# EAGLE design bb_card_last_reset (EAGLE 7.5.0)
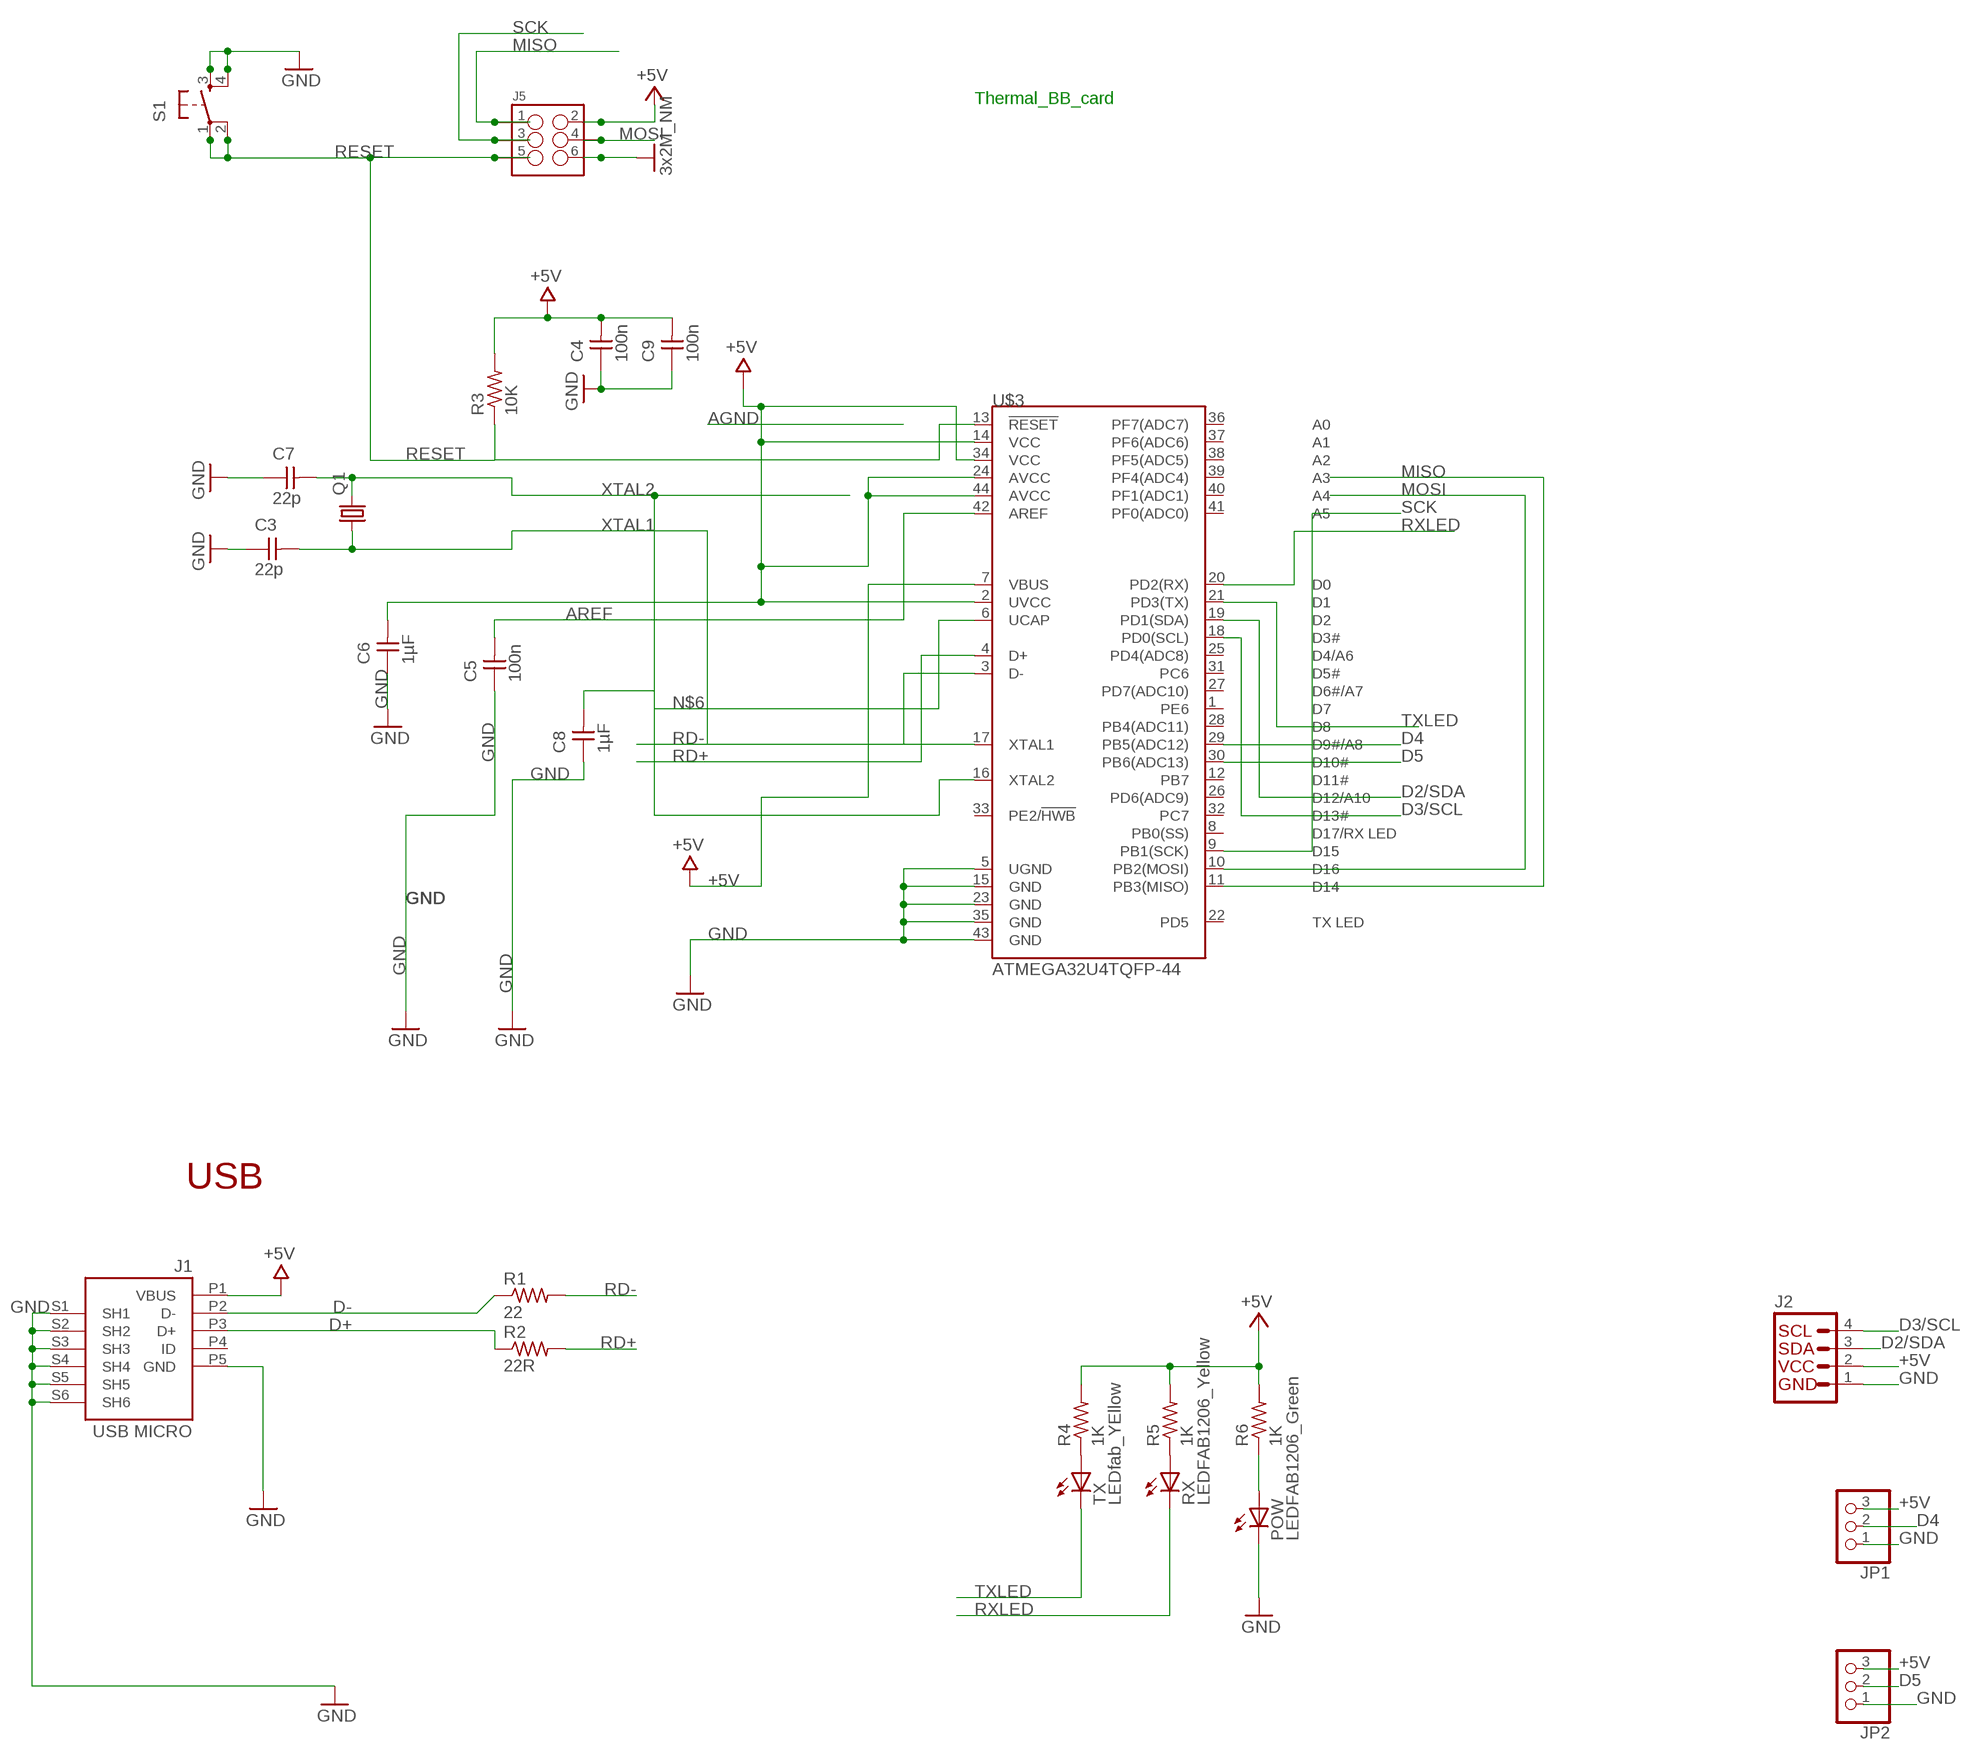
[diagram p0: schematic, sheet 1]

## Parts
C3  22p  CAP-UNPOLARIZEDFAB  [C1206FAB]
C4  100n  CAP-UNPOLARIZEDFAB  [C1206FAB]
C5  100n  CAP-UNPOLARIZEDFAB  [C1206FAB]
C6  1µF  CAP-UNPOLARIZEDFAB  [C1206FAB]
C7  22p  CAP-UNPOLARIZEDFAB  [C1206FAB]
C8  1µF  CAP-UNPOLARIZEDFAB  [C1206FAB]
C9  100n  CAP-UNPOLARIZEDFAB  [C1206FAB]
J1  USB MICRO  MYCON2_USB-MINI-B  [CON2_USB_MICRO_B_AT]
J2  I2C_STANDARD  [1X04]
J5  M03X2  [2X3_SMD]
JP1  PINHD-1X3  [1X03]
JP2  PINHD-1X3  [1X03]
POW  LEDFAB1206_Green  LEDFAB1206  [LED1206FAB]
Q1  CRYSTALHC49UP  [HC49UP]
R1  22  RES-US1206FAB  [R1206FAB]
R2  22R  RES-US1206FAB  [R1206FAB]
R3  10K  RES-US1206FAB  [R1206FAB]
R4  1K  RES-US1206FAB  [R1206FAB]
R5  1K  RES-US1206FAB  [R1206FAB]
R6  1K  RES-US1206FAB  [R1206FAB]
RX  LEDFAB1206_Yellow  LEDFAB1206  [LED1206FAB]
S1  6MM_SWITCH6MM_SWITCH  [6MM_SWITCH]
TX  LEDfab_YEllow  LEDFAB1206  [LED1206FAB]
U$3  ATMEGA32U4TQFP-44  [TQFP44]

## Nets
+5V [usbvcc]: C4.2 C6.2 C9.2 J1.P1(VBUS) J2.2 J5.2 JP1.3 JP2.3 R3.2 R4.2 R5.2 R6.2 U$3.2(UVCC) U$3.7(VBUS) U$3.14(VCC) U$3.24(AVCC) U$3.34(VCC) U$3.44(AVCC)
AREF [aref]: C5.2 U$3.42(AREF)
D2/SDA: J2.3 U$3.19(PD1(SDA))
D3/SCL: J2.4 U$3.18(PD0(SCL))
D4: JP1.2 U$3.29(PB5(ADC12))
D5: JP2.2 U$3.30(PB6(ADC13))
D+: J1.P3(D+) R2.1
D-: J1.P2(D-) R1.1
GND [gnd]: C3.1 C4.1 C5.1 C6.1 C7.1 C8.1 C9.1 J1.P5(GND) J1.S1(SH1) J1.S2(SH2) J1.S3(SH3) J1.S4(SH4) J1.S5(SH5) J1.S6(SH6) J2.1 J5.6 JP1.1 JP2.1 POW.2(C) S1.3(S) S1.4(S1) U$3.5(UGND) U$3.15(GND) U$3.23(GND) U$3.35(GND) U$3.43(GND) ; supply symbol labelled 3x2M_NM
MISO: J5.1 U$3.11(PB3(MISO))
MOSI: J5.4 U$3.10(PB2(MOSI))
N$1: R4.1 TX.1(A)
N$2: R5.1 RX.1(A)
N$3: POW.1(A) R6.1
N$6: C8.2 U$3.6(UCAP)
RD+: R2.2 U$3.4(D+)
RD-: R1.2 U$3.3(D-)
RESET: J5.5 R3.1 S1.1(P) S1.2(P1) U$3.13(!RESET)
RXLED: RX.2(C) U$3.20(PD2(RX))
SCK: J5.3 U$3.9(PB1(SCK))
TXLED: TX.2(C) U$3.21(PD3(TX))
XTAL1: C3.2 Q1.1 U$3.17(XTAL1)
XTAL2: C7.2 Q1.2 U$3.16(XTAL2)
Unconnected: J1.P4(ID) U$3.1(PE6) U$3.8(PB0(SS)) U$3.12(PB7) U$3.22(PD5) U$3.25(PD4(ADC8)) U$3.26(PD6(ADC9)) U$3.27(PD7(ADC10)) U$3.28(PB4(ADC11)) U$3.31(PC6) U$3.32(PC7) U$3.33(PE2/!HWB) U$3.36(PF7(ADC7)) U$3.37(PF6(ADC6)) U$3.38(PF5(ADC5)) U$3.39(PF4(ADC4)) U$3.40(PF1(ADC1)) U$3.41(PF0(ADC0))

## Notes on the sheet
- Thermal_BB_card
- USB

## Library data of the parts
C3-C9 = fab (1):CAP-UNPOLARIZED
J1 = SmartPrj:MYCON2_USB-MINI-B
J2 = SparkFun-Connectors:I2C_STANDARD: SparkFun has standardized on a pinout for all I2C based sensor breakouts. This pinout allows I2C boards to be plugged directly into the headers on Arduino Uno compatible boards, and to be daisy chained easily.
J5 = SparkFun-Connectors:M03X2: 2x3 .1" header. Shrouded, with keying- CONN-10681 SMT- CONN-11415 Pogo pins- HW-11044; PROD_ID: CONN-11290
JP1 JP2 = pinhead:PINHD-1X3: PIN HEADER
POW RX TX = fab (1):LED: LED
Q1 = crystal:CRYSTAL: CRYSTAL; OC_FARNELL: unknown; OC_NEWARK: unknown
R1-R6 = fab (1):RES-US: Resistor (US Symbol)
S1 = fab (1):6MM_SWITCH: OMRON SWITCH
U$3 = SparkFun-DigitalIC:ATMEGA32U4: Atmel 44-pin 8-bit Microcontroller with 32KBytes of ISP Flash and USB Controller

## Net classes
0 default: width 0.254 mm, drill 0.61 mm, clearance 0.254 mm
1 power: width 0.254 mm, drill 0.61 mm, clearance 0.254 mm
2 gnd: width 0.254 mm, drill 0.61 mm, clearance 0.254 mm
3 usbvcc: width 0.254 mm, drill 0.61 mm, clearance 0.254 mm
4 aref: width 0.254 mm, drill 0.61 mm, clearance 0.254 mm

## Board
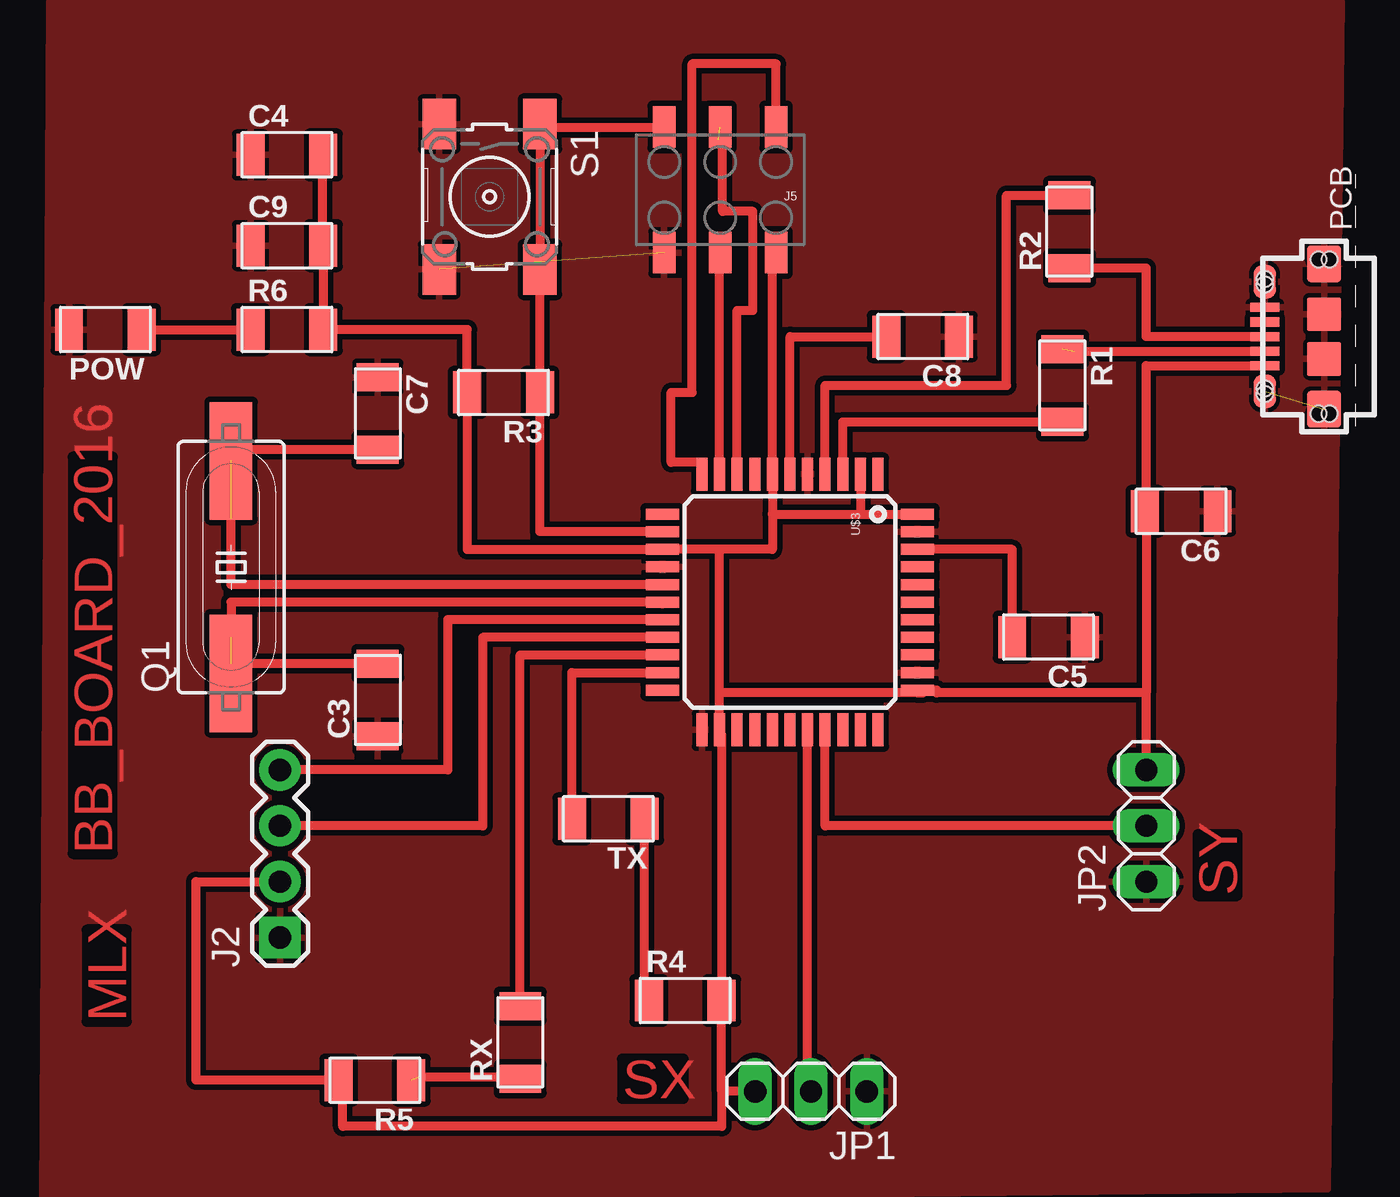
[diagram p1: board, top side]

No outline drawn. Coordinates in mm, seen from the top.
Copper layers (1*16): Top 0.018mm / dielectric 1.55mm / Bottom 0.018mm
Design rules "eC_2Layer_PClass6_BaseCopperO18_eCDefault *": minimum track width 0.15mm, minimum drill 0.35mm, track to track 0.01mm, track to pad 0.01mm, pad to pad 0.01mm, via to via 0.15mm, smd to smd 0mil, copper to edge 0.25mm, drill to drill 0.35mm, minimum pad ring 0.175mm, minimum via ring 0.125mm, stop-mask expansion 0mil, vias tented up to drill 0.45mm, thermal gap 0.2mm

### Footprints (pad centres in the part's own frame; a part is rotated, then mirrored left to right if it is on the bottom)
C1206FAB = smd 1.27 x 1.905: 1 -1.651,0; 2 1.651,0
CON2_USB_MICRO_B_AT = smd 0.406 x 1.346: P1 -1.321,2.692; P2 -0.66,2.692; P3 0,2.692; P4 0.66,2.692; P5 1.321,2.692 | smd 1.651 x 1.549: S1 -3.302,0; S2 3.302,0 | smd 1.524 x 1.016: S3 -2.489,2.692; S4 2.489,2.692 | smd 1.524 x 1.524: S5 -1.016,0; S6 1.016,0 | hole 0.7: -3.505,0.254; -3.505,-0.254; 3.505,0.254; 3.505,-0.254; -2.616,2.692; -2.362,2.692; 2.362,2.692; 2.616,2.692
1X04 = drill 1.016 pad 1.88 square: 1 0,0 | drill 1.016 pad 1.88: 2 2.54,0; 3 5.08,0; 4 7.62,0
2X3_SMD = smd 1.02 x 1.9: 1 -2.54,-2.85; 2 -2.54,2.85; 3 0,-2.85; 4 0,2.85; 5 2.54,-2.85; 6 2.54,2.85
1X03 = drill 1.016 long: 1 -2.54,0; 2 0,0; 3 2.54,0
LED1206FAB = smd 1.27 x 1.905: 1 -1.651,0; 2 1.651,0
HC49UP = smd 5.334 x 1.93: 1 -4.826,0; 2 4.826,0
R1206FAB = smd 1.27 x 1.905: 1 -1.651,0; 2 1.651,0
6MM_SWITCH = smd 2.286 x 1.524: 1 -3.302,2.286; 2 3.302,2.286; 3 -3.302,-2.286; 4 3.302,-2.286
TQFP44 = smd 1.5 x 0.5: 1 -5.8,4; 2 -5.8,3.2; 3 -5.8,2.4; 4 -5.8,1.6; 5 -5.8,0.8; 6 -5.8,0; 7 -5.8,-0.8; 8 -5.8,-1.6; 9 -5.8,-2.4; 10 -5.8,-3.2; 11 -5.8,-4; 23 5.8,-4; 24 5.8,-3.2; 25 5.8,-2.4; 26 5.8,-1.6; 27 5.8,-0.8; 28 5.8,0; 29 5.8,0.8; 30 5.8,1.6; 31 5.8,2.4; 32 5.8,3.2; 33 5.8,4 | smd 0.5 x 1.5: 12 -4,-5.8; 13 -3.2,-5.8; 14 -2.4,-5.8; 15 -1.6,-5.8; 16 -0.8,-5.8; 17 0,-5.8; 18 0.8,-5.8; 19 1.6,-5.8; 20 2.4,-5.8; 21 3.2,-5.8; 22 4,-5.8; 34 4,5.8; 35 3.2,5.8; 36 2.4,5.8; 37 1.6,5.8; 38 0.8,5.8; 39 0,5.8; 40 -0.8,5.8; 41 -1.6,5.8; 42 -2.4,5.8; 43 -3.2,5.8; 44 -4,5.8

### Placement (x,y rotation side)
C3  35.56,33.02 90 top
C4  31.43,57.78 0 top
C5  66.04,35.88 180 top
C6  72.07,41.59 180 top
C7  35.56,46.04 270 top
C8  60.33,49.53 180 top
C9  31.43,53.66 0 top
J1  78.56,49.53 90 top
J2  31.11,22.23 90 top
J5  51.12,56.2 180 top
JP1  55.24,15.24 180 top
JP2  70.48,27.3 90 top
POW  23.18,49.85 180 top
Q1  28.89,39.05 90 top
R1  66.67,47.31 270 top
R2  66.99,54.29 90 top
R3  41.27,46.99 180 top
R4  49.53,19.37 0 top
R5  35.43,15.75 180 top
R6  31.43,49.85 0 top
RX  42.04,17.46 90 top
S1  40.64,55.88 270 top
TX  46.04,27.62 180 top
U$3  54.29,37.47 270 top

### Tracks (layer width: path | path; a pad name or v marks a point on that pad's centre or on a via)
+5V
  Top 0.406: JP1.3 51.18,15.24 | 51.18,15.24 R4.2 51.18,31.43 51.12,31.43 51.12,31.66 U$3.24 51.09,33.34 | J2.2 27.3,24.77 27.3,15.75 R5.2 33.97,15.75 33.97,13.65 51.18,13.65 51.18,15.24 | R6.2 33.02,49.85 | C4.2 33.02,57.78 33.02,53.66 C9.2 R6.2 | JP2.3 70.48,33.34 | 70.48,33.34 60.96,33.34 60.96,33.47 U$3.34 60.09,33.34 | 70.17,41.59 C6.2 70.48,41.59 | 70.48,41.59 70.48,33.34 | 70.48,41.59 70.48,48.21 J1.P1 | 53.49,41.47 U$3.7 53.49,53.35 J5.2 | 53.49,41.47 57.49,41.47 | 57.49,41.47 U$3.44 | 53.49,41.47 53.49,39.87 51.09,39.87 | 51.09,39.87 U$3.14 39.62,39.87 R3.2 39.62,49.85 R6.2 | 51.09,33.34 51.09,39.87 | U$3.2 57.49,41.47 | 60.09,33.34 60.33,33.34 | 60.09,33.34 51.09,33.34
AREF
  Top 0.406: C5.2 64.39,39.87 U$3.42
D2/SDA
  Top 0.406: U$3.19 40.32,35.87 40.32,27.3 J2.3
D3/SCL
  Top 0.406: U$3.18 38.73,36.66 38.73,29.84 J2.4
D4
  Top 0.406: JP1.2 55.09,15.24 U$3.29
D5
  Top 0.406: JP2.2 55.89,27.3 U$3.30
D+
  Top 0.406: J1.P3 70.48,49.53 70.48,52.64 R2.1
D-  (1 unrouted)
  Top 0.406: J1.P2 75.87,48.84 67.21,48.84
GND  (3 unrouted)
  pour Top: 78.74,10.79 79.38,64.77 20.64,64.77 20.32,10.16
MISO
  Top 0.406: U$3.11 50.29,43.81 48.9,43.81 48.9,46.99 49.85,46.99 49.85,61.91 53.66,61.91 J5.1
MOSI
  Top 0.406: U$3.10 51.09,53.35 J5.4
N$1
  Top 0.406: R4.1 47.69,19.37 TX.1
N$2  (1 unrouted)
  Top 0.406: RX.1 42.04,15.88 37.47,15.88
N$3
  Top 0.406: POW.1 R6.1
N$6
  Top 0.406: U$3.6 54.29,49.53 C8.2
RD+
  Top 0.406: U$3.4 55.89,47.31 64.14,47.31 64.14,55.94 R2.2
RD-
  Top 0.406: U$3.3 56.69,45.66 R1.2
RESET
  Top 0.406: U$3.13 42.93,40.66 R3.1 S1.2 42.93,59.05 42.86,59.05 42.86,59.18 S1.1 42.93,59.05 J5.5
RXLED
  Top 0.406: RX.2 42.04,35.06 U$3.20
SCK  (1 unrouted)
  Top 0.406: U$3.9 51.89,50.72 52.6,50.72 52.6,55.22 51.23,55.22 51.23,58.47 51.05,58.47
TXLED
  Top 0.406: TX.2 44.39,34.27 U$3.21
XTAL1  (1 unrouted)
  Top 0.406: 48.49,37.37 U$3.17 28.89,37.47 28.89,35.88 | C3.2 28.89,34.67 Q1.1
XTAL2  (1 unrouted)
  Top 0.406: U$3.16 28.89,38.27 28.89,41.27 | C7.2 28.89,44.39 Q1.2

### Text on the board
Top: BB_BOARD_2016 | SY | MLX | SX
